[IBIS ver]   3.2
[File name]   sprm202c.ibs
[File Rev]   1.0
[Date]   August 11, 2005
[Source]   TI
[Disclaimer]   Please be aware that in the absence of a written agreement
|   Texas Instruments(TI) assumes no liability for:
|   (1) The accuracy of the IBIS models provided to your company
|   (2) The proper functioning of these Models in your design
|   or for any resulting applications
|   (3) Infringement of patents, copyrights or intellectual
|   property rights resulting from your use of these
|   models.
|   TI provides IBIS Models as a service to our customers and
|   therefore reserves the right to limit distribution of the
|   Models.
[Copyright]   Property of Texas Instruments Incorporated.
|   Unauthorized reproduction and/or distribution is strictly.
|   prohibited.
|   This product is protected under copyright law and trade
|   secret law as an unpublished work.
|   Created 2003,(C) Copyright 1999-2003,
|   Texas Instruments Incorporated., All Rights Reserved.
|   These commodities are under the U.S. Government
|   distribution license control. As such,they are not to be
|   re-exported without the prior approval of the U.S.
|   Department of Commerce.
[Notes]   See individual buffer models for additional notes.
|****** ****   ***** *****   ******  Package Model  ***************************
[Component]   DAVINCI_ZWT
[Manufacturer]  Texas Instruments
[Package]
|variable   typ   min   max
R_pkg   0.30489   0.23517194   0.41076
L_pkg   4.09242n   2.12433n   9.57717n
C_pkg   1.20919p   1.16455p   1.41723p
[Pin] signal_name   model_name   R_pin   L_pin   C_pin
K17  YI1_CCD1   BC1850BSHYPDFZ   0.27142   3.26611n   1.24171p
E11  GIOV3310_RXD3   BT3350BSHYPDFZP18_Z 0.26648   3.27345n   1.21648p
D8   SD_DATA0   BT3350BSHYPDFZP18_Z 0.26424   3.13901n   1.23471p
C11  GIOV338_RXD1   BT3350BSHYPDFZP18_Z 0.32683   4.77147n   1.21112p
E4   EMD4_DD4   BC1850BSHYPDFZ_PDZ  0.24370885  2.59914n   1.25295p
N19  CI7_CCD15_UARTRXD2   BC1850BSHYPDFZ   0.32265   4.61826n   1.18113p
N18  CI6_CCD1_UARTTXD2   BC1850BSHYPDFZ   0.30424   3.95206n   1.18245p
N17  CI5_CCD13_UARTCTS2   BC1850BSHYPDFZ   0.23966353  2.25930n   1.17595p
N15  CI3_CCD11   BC1850BSHYPDFZ   0.25136   2.72422n   1.21653p
M15  CI0_CCD8   BC1850BSHYPDFZ   0.23948995  2.24177n   1.1961p
N16  CI4_CCD12_UARTRTS2   BC1850BSHYPDFZ   0.32117   4.53767n   1.23269p
M17  CI2_CCD10   BC1850BSHYPDFZ   0.29397   3.52173n   1.18996p
M16  CI1_CCD9   BC1850BSHYPDFZ   0.29839   3.66820n   1.19339p
M19  PCLK   BC1850BSHYPDFZ_PDZ  0.32124   4.54005n   1.16939p
L19  VD   BC1850BSHYPDFZ_PDZ  0.32051   4.55204n   1.17582p
M18  HD   BC1850BSHYPDFZ_PDZ  0.30044   3.73376n   1.16728p
L18  YI7_CCD7   BC1850BSHYPDFZ   0.30158   3.82514n   1.17562p
L17  YI6_CCD6   BC1850BSHYPDFZ   0.24008563  2.27632n   1.175p
L16  YI5_CCD5   BC1850BSHYPDFZ   0.31818   4.44138n   1.22761p
L15  YI4_CCD4   BC1850BSHYPDFZ   0.25554   2.83961n   1.21082p
K19  YI3_CCD3   BC1850BSHYPDFZ   0.3193   4.49825n   1.17099p
K18  YI2_CCD2   BC1850BSHYPDFZ   0.30113   3.80508n   1.17045p
K16  YI0_CCD0   BC1850BSHYPDFZ   0.29716   3.67499n   1.19867p
E19  CLKOUT1_TIMIN_GPIO49   BC1850BSHYPDFZ_PDZ  0.34024   5.31946n   1.20264p
E15  YOUT4_R4_AEAW4   BC1850BSHYPDFZ   0.34642   5.54214n   1.30793p
E16  YOUT5_R5   BC1850BSHYPDFZ_PDZ  0.32347   4.68532n   1.28314p
D19  VCLK   BC1850BSHYPDFZ_PDZ  0.34898   5.65973n   1.2157p
C19  VPBECLK   BC1850BSHYPDFZ   0.35532   5.90192n   1.225p
B19  COUT6_G3   BC1850BSHYPDFZ_PDZ  0.36768   6.39976n   1.24506p
E18  YOUT7_R7   BC1850BSHYPDFZ_PDZ  0.30638   4.04896n   1.24212p
E17  YOUT6_R6   BC1850BSHYPDFZ_PDZ  0.30907   4.16196n   1.28916p
D15  YOUT0_G5_AEAW0   BC1850BSHYPDFZ   0.3463   5.62598n   1.37049p
D16  YOUT1_G6_AEAW1   BC1850BSHYPDFZ   0.31601   5.21148n   1.33301p
C16  COUT7_G4   BC1850BSHYPDFZ_PDZ  0.3081   4.99577n   1.34461p
D18  YOUT3_R3_AEAW3   BC1850BSHYPDFZ   0.31075   4.22512n   1.2403p
C18  VSYNC   BC1850BSHYPDFZ   0.31724   4.48625n   1.23593p
B18  COUT5_G2   BC1850BSHYPDFZ_PDZ  0.33021   4.96230n   1.23197p
C17  HSYNC   BC1850BSHYPDFZ   0.30581   4.10873n   1.2456p
D17  YOUT2_G7_AEAW2   BC1850BSHYPDFZ   0.30617   4.87215n   1.28815p
B17  COUT3_B6_DSPBT   BC1850BSHYPDFZ   0.329   4.61176n   1.20617p
A18  COUT4_B7   BC1850BSHYPDFZ_PDZ  0.33688   4.93706n   1.20091p
B16  COUT1_B4_BTSEL1   BC1850BSHYPDFZ   0.30834   3.87063n   1.19717p
A17  COUT2_B5_EMWIDTH   BC1850BSHYPDFZ   0.32513   4.53204n   1.19667p
C15  PWM0_GPIO45   BC1850BSHYPDFZ_PDZ  0.25161   2.59187n   1.20447p
B15  PWM1_R2_GPIO46   BC1850BSHYPDFZ_PDZ  0.31665   4.23770n   1.19062p
E14  GPIO5_G1   BC1850BSHYPDFZ_PDZ  0.25976   2.88215n   1.22562p
A16  COUT0_B3_BTSEL0   BC1850BSHYPDFZ   0.33512   4.91629n   1.18803p
P5   EMA18_GIO13_VLNQRXD1   BC1850BSHYPDFZ_PDZ  0.25928   3.04090n   1.26652p
R5   EMA16_GIO15_VLNQRXD2   BC1850BSHYPDFZ_PDZ  0.2672   3.33832n   1.25638p
T2   EMCS4_GIO9_VLNQSCRUN   BC1850BSHYPDFZ_PDZ  0.29472   3.50721n   1.18161p
T1   EMCS5_GIO8_VLNQCLOCK   BC1850BSHYPDFZ_PDZ  0.30976   4.10843n   1.1798p
T3   EMA21_GIO10_VLNQTXD0   BC1850BSHYPDFZ_PDZ  0.29934   3.81398n   1.21837p
R4   EMA19_GIO12_VLNQTXD1   BC1850BSHYPDFZ_PDZ  0.30272   3.86488n   1.21797p
N4   EMA13_GPIO18   BC1850BSHYPDFZ_PDZ  0.23736136  2.17244n   1.21241p
R3   EMA20_GIO11_VLNQRXD0   BC1850BSHYPDFZ_PDZ  0.29279   3.54781n   1.20942p
R2   EMA17_GIO14_VLNQTXD2   BC1850BSHYPDFZ_PDZ  0.30435   3.91825n   1.18246p
P3   EMA15_GIO16_VLNQTXD3   BC1850BSHYPDFZ_PDZ  0.29342   3.47425n   1.20306p
P4   EMA14_GIO17_VLNQRXD3   BC1850BSHYPDFZ_PDZ  0.29742   3.72080n   1.22221p
R1   EMA12_GPIO19   BC1850BSHYPDFZ_PDZ  0.33141   4.91831n   1.18807p
P1   EMA10_GPIO21   BC1850BSHYPDFZ_PDZ  0.32107   4.51855n   1.17303p
P2   EMA11_GPIO20   BC1850BSHYPDFZ_PDZ  0.30527   3.92717n   1.1797p
N3   EMA8_GPIO23   BC1850BSHYPDFZ_PDZ  0.29205   3.40450n   1.18847p
L4   RESETN   IC18SHYPUFZ   0.24060459  2.27896n   1.19435p
M4   EMA9_GPIO22   BC1850BSHYPDFZ_PDZ  0.23754022  2.16867n   1.17725p
N1   EMA6_GPIO25   BC1850BSHYPDFZ_PDZ  0.32162   4.52466n   1.17019p
K1   CLKOUT0_GPIO48   BC1850BSHYPDFZ_PDZ  0.30266   3.85884n   1.17499p
L1   CLKIN   IOSCHF18SHY   0.31844   4.39342n   1.16471p
K4   EMA4_GPIO27   BC1850BSHYPDFZ_PDZ  0.32093   4.55345n   1.22883p
J5   GPIO50_ATACS0   BC1850BSHYPDFZ_PDZ  0.25488   2.84503n   1.21689p
J4   EMA0_DA2_GPIO53   BC1850BSHYPDFZ_PDZ  0.23939151  2.29806n   1.18231p
J3   EMBA0_DA0   BC1850BSHYPDFZ_PDZ  0.2359258   2.13113n   1.17721p
K3   EMA5_GPIO26   BC1850BSHYPDFZ_PDZ  0.29597   3.55241n   1.18676p
K2   EMA3_GPIO28   BC1850BSHYPDFZ_PDZ  0.29881   3.67469n   1.16455p
J1   EMA2   BC1850BSHYPDFZ_PDZ  0.3178   4.41430n   1.16743p
H3   DMACK_UARTTXD1   BC1850BSHYPDFZ_PDZ  0.28904   3.34897n   1.19571p
H1   GPIO51_ATACS1   BC1850BSHYPDFZ_PDZ  0.31476   4.31632n   1.16847p
J2   EMA1   BC1850BSHYPDFZ_PDZ  0.29951   3.72938n   1.16729p
H2   EMBA1_DA1_GPIO52   BC1850BSHYPDFZ_PDZ  0.30016   3.76002n   1.16876p
G1   DMARQ_UARTRXD1   BC1850BSHYPDFZ   0.32209   4.59886n   1.17782p
D14  GPIO38_R1   BC1850BSHYPDFZ_PDZ  0.24943373  2.49462n   1.19177p
E13  GPIO1_CWE   BC1850BSHYPDFZ_PDZ  0.24702782  2.38582n   1.20009p
D13  GPIO2_G0   BC1850BSHYPDFZ_PDZ  0.24580039  2.35534n   1.19321p
D12  GIOV334_TXD1   BT3350BSHYPDFZP18_Z 0.25534   2.76733n   1.21955p
E12  GIOV337_RXD0   BT3350BSHYPDFZP18_Z 0.25098   2.49201n   1.21562p
E10  GIOV3315_MDIO   BT3350BSHYPDFZP18_Z 0.25609   2.68714n   1.21016p
E9   SD_DATA1   BT3350BSHYPDFZP18_Z 0.26906   3.20966n   1.23725p
A15  PWM2_B2_GPIO47   BC1850BSHYPDFZ_PDZ  0.33245   4.82511n   1.18357p
A14  GPIO6_B1   BC1850BSHYPDFZ_PDZ  0.33354   4.86754n   1.18579p
B14  GPIO4_R0_CFIELD   BC1850BSHYPDFZ_PDZ  0.31277   4.12134n   1.1868p
C14  GPIO3_B0_LCDFIELD   BC1850BSHYPDFZ_PDZ  0.29883   3.54970n   1.19368p
C13  GPIO0_LCDOE   BC1850BSHYPDFZ_PDZ  0.30633   3.83629n   1.20463p
C12 GIOV336_TXD3   BT3350BSHYPDFZP18_Z 0.30666   3.80383n   1.20363p
A11 GIOV335_TXD2   BT3350BSHYPDFZP18_Z 0.33469   4.95163n   1.19018p
A12 GIOV332_COL   BT3350BSHYPDFZP18_Z 0.32801   4.64818n   1.17868p
A13 GIOV331_TXCLK   BT3350BSHYPDFZP18_Z 0.31242   4.05710n   1.17723p
B13 GIOV330_TXEN   BT3350BSHYPDFZP18_Z 0.30624   3.82421n   1.17796p
B12 GIOV333_TXD0   BT3350BSHYPDFZP18_Z 0.31117   4.04273n   1.18423p
B11 GIOV339_RXD2   BT3350BSHYPDFZP18_Z 0.31218   4.00065n   1.17507p
A10 GIOV3311_RXCLK   BT3350BSHYPDFZP18_Z 0.33193   4.78827n   1.18217p
D11 GIOV3312_RXDV   BT3350BSHYPDFZP18_Z 0.31026   3.93739n   1.20497p
D10 GIOV3313_RXER   BT3350BSHYPDFZP18_Z 0.31235   4.09340n   1.21604p
C10 GIOV3314_CRS   BT3350BSHYPDFZP18_Z 0.31221   3.99279n   1.2065p
B10 GIOV3316_MDCLK   BT3350BSHYPDFZP18_Z 0.31256   4.00376n   1.17687p
C9  SD_DATA3   BT3350BSHYPDFZP18_Z 0.31135   3.97934n   1.20841p
A9  SD_CLK   BT3350BSHYPDFZP18_Z 0.33142   4.72337n   1.17817p
B9  SD_CMD   BT3350BSHYPDFZP18_Z 0.31656   4.20830n   1.18471p
D9  SD_DATA2   BT3350BSHYPDFZP18_Z 0.31824   4.24185n   1.21905p
C8  FSX_GIO31   BC1850BSHYPDFZ_PDZ  0.31499   4.10649n   1.21449p
B8  CLKX_GPIO29   BC1850BSHYPDFZ_PDZ  0.31718   4.24766n   1.18779p
A8  CLKR_GPIO30   BC1850BSHYPDFZ_PDZ  0.32026   4.30407n   1.18253p
F5  EMD2_DD2   BC1850BSHYPDFZ_PDZ  0.24446141  2.54036n   1.26565p
D7  NTRST   IC18SHYPDFZ   0.25102   2.57722n   1.20656p
D6  EMU0   BC1850BSHYPUFZ   0.26369   3.00542n   1.22142p
E6  TMS   IC18SHYPUFZ   0.26016   2.89933n   1.23079p
D5  UARTRXD0_GPIO35   BC1850BSHYPDFZ_PDZ  0.32087   4.37168n   1.23559p
C3  GPIO7   BC1850BSHYPDFZ_PDZ  0.28444   3.81897n   1.26078p
H5  EMD14_DD14   BC1850BSHYPDFZ_PDZ  0.25134   2.74799n   1.2613p
G5  EMD10_DD10   BC1850BSHYPDFZ_PDZ  0.24763525  2.62779n   1.25179p
H4  EMOE_DIOR   BC1850BSHYPDFZ_PDZ  0.23517194  2.12433n   1.183p
G3  EMRNW_INTRQ   BC1850BSHYPDFZ_PDZ  0.24110686  2.36803n   1.22429p
F4  EMD6_DD6   BC1850BSHYPDFZ_PDZ  0.23553426  2.20052n   1.22333p
G2  EMWE_DIOW   BC1850BSHYPDFZ_PDZ  0.3026   3.92018n   1.18023p
F1  EMWAIT_IORDY   BC1850BSHYPUFZ   0.32084   4.57333n   1.17696p
E1  EMD15_DD15   BC1850BSHYPDFZ_PDZ  0.33258   5.06281n   1.19705p
F2  EMD13_DD13   BC1850BSHYPDFZ_PDZ  0.30858   4.20967n   1.20886p
D1  EMD12_DD12   BC1850BSHYPDFZ_PDZ  0.34172   5.41604n   1.2124p
G4  EMD11_DD11   BC1850BSHYPDFZ_PDZ  0.29109   3.46731n   1.23452p
F3  EMD8_DD8   BC1850BSHYPDFZ_PDZ  0.28411   3.21952n   1.22681p
E2  EMD9_DD9   BC1850BSHYPDFZ_PDZ  0.30321   3.93813n   1.21141p
C1  EMD7_DD7   BC1850BSHYPDFZ_PDZ  0.34316   5.47607n   1.21459p
D2  EMD5_DD5   BC1850BSHYPDFZ_PDZ  0.30837   4.15257n   1.21424p
E5  EMD0_DD0   BC1850BSHYPDFZ_PDZ  0.23865047  2.31435n   1.2451p
E3  EMD3_DD3   BC1850BSHYPDFZ_PDZ  0.28366   3.21871n   1.22369p
D3  EMD1_DD1   BC1850BSHYPDFZ_PDZ  0.2921   3.60704n   1.24282p
C7  FSR_GPIO32   BC1850BSHYPDFZ_PDZ  0.31555   4.22094n   1.21883p
A7  DR_GPIO34   BC1850BSHYPDFZ_PDZ  0.32996   4.67616n   1.17937p
C6  EMU1   BC1850BSHYPUFZ   0.3118   4.01559n   1.20949p
B7  DX_GPIO33   BC1850BSHYPDFZ_PDZ  0.31643   4.22763n   1.18564p
A6  TCK   IC18SHYPUFZ   0.3335   4.85058n   1.1798p
B5  TDO   OC1850BSFZ   0.32041   4.41194n   1.19295p
A5  TDI   IC18SHYPUFZ   0.33719   4.99894n   1.18952p
C4  SCL_GPIO43   BC1850BSHYPDFZ_PDZ  0.31456   4.20146n   1.23233p
C5  UARTTXD0_GPIO38   BC1850BSHYPDFZ_PDZ  0.30441   3.82552n   1.21979p
B4  SDA_GPIO44   BC1850BSHYPDFZ_PDZ  0.32308   4.45433n   1.19164p
B6  RTCK   OC1850BSFZ   0.31193   4.03099n   1.17724p
A3  SPICLK_GPIO39   BC1850BSHYPDFZ_PDZ  0.33139   4.77785n   1.19765p
B3  SPIDI_GPIO40   BC1850BSHYPDFZ_PDZ  0.32391   4.48887n   1.20374p
A4  SPIEN0_GPIO37   BC1850BSHYPDFZ_PDZ  0.34182   5.15828n   1.19449p
B2  SPIEN1_GPIO42   BC1850BSHYPDFZ_PDZ  0.33542   4.91202n   1.21886p
A2  SPIDO_GPIO41   BC1850BSHYPDFZ_PDZ  0.34148   5.16190n   1.21506p
B1  EM_CS3   BC1850BSHYPDFZ_PDZ  0.34927   5.38565n   1.22986p
C2  EM_CS2   BC1850BSHYPDFZ_PDZ  0.3251   4.50591n   1.22482p
N2  EMA7_GPIO24   BC1850BSHYPDFZ_PDZ  0.30209   3.80241n   1.17344p
|****** ****   ***** *****   ******  Buffer Models  ***************************
|   Component BC1850BSHYPDFZ
|[Notes]   Driver/Receiver, CMOS, 1.8 V, 50 ohms, Fnom < 100 MHz,
|   min-height, non-failsafe, hysteresis, pulldown, with HHV
[Component]   BC1850BSHYPDFZ
[Manufacturer]   Texas Instruments.
[Package]
| variable   typ   min   max
R_pkg   0.000   0.000   0.000
L_pkg   0.000H   0.000H   0.000H
C_pkg   0.000F   0.000F   0.000F
[Pin]  signal_name   model_name   R_pin   L_pin   C_pin
1   PAD   BC1850BSHYPDFZ
|2   A   (input)
|3   GZ   (Driver enable)
|4   HHV   (force Z)
|5   PI   (pulldown Inhibit)
|6   Y   (receiver output)
|7   VDD   (1.2V core supply)
8   VDDS   POWER
9   VSS   GND
10   VSSS   GND
[Model Selector]   BC1850BSHYPDFZ
BC1850BSHYPDFZ_1P8PD   Cell operated at VDDS=1.8V(nom) with pulldown "on"
BC1850BSHYPDFZ_PDZ   Cell operated at VDDS=1.8V(nom) with pulldown "off"
|   Component BC1850BSHYPUFZ
|[Notes]   Driver/Receiver, CMOS, 1.8 V, 50 ohms, Fnom < 100 MHz,
|   min-height, non-failsafe, hysteresis, pull-up, with HHV
[Component]   BC1850BSHYPUFZ
[Manufacturer]   Texas Instruments.
[Package]
| variable   typ   min   max
R_pkg   0.000   0.000   0.000
L_pkg   0.000H   0.000H   0.000H
C_pkg   0.000F   0.000F   0.000F
[Pin]  signal_name   model_name   R_pin   L_pin   C_pin
1   PAD   BC1850BSHYPUFZ
|2   A   (input)
|3   GZ   (Driver enable)
|4   HHV   (force Z)
|5   PI   (pullup Inhibit)
|6   Y   (receiver output)
|7   VDD   (1.2V core supply)
8   VDDS   POWER
9   VSS   GND
10   VSSS   GND
[Model Selector]   BC1850BSHYPUFZ
BC1850BSHYPUFZ_PU   Cell operated at VDDS=1.8V(nom) with Pullup "on"
BC1850BSHYPUFZ_PUZ   Cell operated at VDDS=1.8V(nom) with Pullup "off"
|   Component BC1850CSHYPDFZ
|[Notes]   Driver/Receiver, CMOS, 1.8 V, 50 ohms, Fnom < 150 MHz,
|   min-height, non-failsafe,hysteresis, pulldown, with HHV
[Component]   BC1850CSHYPDFZ
[Manufacturer]   Texas Instruments.
[Package]
| variable   typ   min   max
R_pkg   0.000   0.000   0.000
L_pkg   0.000H   0.000H   0.000H
C_pkg   0.000F   0.000F   0.000F
[Pin]  signal_name   model_name   R_pin   L_pin   C_pin
1   PAD   BC1850CSHYPDFZ
8   VDDS   POWER
9   VSS   GND
10   VSSS   GND
[Model Selector]   BC1850CSHYPDFZ
BC1850CSHYPDFZ_1P8PD   Cell operated at VDDS=1.8V(nom) with pulldown "on"
BC1850CSHYPDFZ_PDZ   Cell operated at VDDS=1.8V(nom) with pulldown "off"
|   Component BT3350BSHYPDFZP18
|[Notes]   Driver/Receiver, TTL, 3.3 V, 50 ohms, Fnom < 100 Mhz,
|   min-height , non-failsafe, hystersis, pull-down
[Component]   BT3350BSHYPDFZP18
[Manufacturer]   Texas Instruments.
[Package]
| variable   typ   min   max
R_pkg   0.000   0.000   0.000
L_pkg   0.000H   0.000H   0.000H
C_pkg   0.000F   0.000F   0.000F
[Pin]  signal_name   model_name   R_pin   L_pin   C_pin
1   PAD   BT3350BSHYPDFZP18
|2   A   (input)
|3   GZ   (Driver enable)
|4   HHV   (Driver tristate)
|5   PI   (pulldown Inhibit)
|6   PWRDN   (low power mode control signal)
|7   Y   (receiver output)
|8   VDD   (1.2V core supply)
9   VDDS   POWER
10   VSS   GND
11   VSSS   GND
[Model Selector]   BT3350BSHYPDFZP18
BT3350BSHYPDFZP18_PD   Cell operated at VDDS=3.3V(nom) with Pulldown "on"
BT3350BSHYPDFZP18_Z   Cell operated at VDDS=3.3V(nom) with Pulldown "off"
|   Component IC18SHYPDFZ
|[Notes]   LVCMOS Receiver, 1.8V, min-height, pullup, HHV control
[Component]   IC18SHYPDFZ
[Manufacturer]   TI
[Package]
| variable   typ   min   max
R_pkg   0.000   0.000   0.000
L_pkg   0.000H   0.000H   0.000H
C_pkg   0.000F   0.000F   0.000F
[Pin]  signal_name   model_name   R_pin   L_pin   C_pin
1   PAD   IC18SHYPDFZ
|2   PI   (Pulldown inhibit)
|3   HHV   (Force Z)
|4   Y   (receiver output)
|5   VDD   (1.2V core supply)
6   VDDS   POWER
7   VSS   GND
[Model Selector]   IC18SHYPDFZ
IC18SHYPDFZ_1P8PD reflects VDDS=1.8V(typ) operation, Pulldown "on"
IC18SHYPDFZ_1P8PDZ reflects VDDS=1.8V(typ) operation, Pulldown "off"
|   Component IC18SHYPUFZ
|[Notes]   LVCMOS Receiver, 1.8V, min-height, pullup, HHV control
[Component]   IC18SHYPUFZ
[Manufacturer]   TI
[Package]
| variable   typ   min   max
R_pkg   0.000   0.000   0.000
L_pkg   0.000H   0.000H   0.000H
C_pkg   0.000F   0.000F   0.000F
[Pin]  signal_name   model_name   R_pin   L_pin   C_pin
1   PAD   IC18SHYPUFZ
|2   PI   (Pullup inhibit)
|3   HHV   (Force Z)
|4   Y   (receiver output)
|5   VDD   (1.2V core supply)
6   VDDS   POWER
7   VSS   GND
[Model Selector]   IC18SHYPUFZ
IC18SHYPUFZ_1P8PU reflects VDDS=1.8V(typ) operation, Pullup "on"
IC18SHYPUFZ_1P8PUZ reflects VDDS=1.8V(typ) operation, Pullup "off"
|   Component OC1850BSFZ
|[Notes]   Driver, CMOS, 1.8 V, 50 ohms, Fnom < 100 MHz, min-height,
|   non-failsafe, with HHV
[Component]   OC1850BSFZ
[Manufacturer]   Texas Instruments.
[Package]
| variable   typ   min   max
R_pkg   0.000   0.000   0.000
L_pkg   0.000H   0.000H   0.000H
C_pkg   0.000F   0.000F   0.000F
[Pin]  signal_name   model_name   R_pin   L_pin   C_pin
1   PAD   OC1850BSFZ
| 2   A   (Driver input)
| 3   GZ   (Driver enable)
| 4   HHV   (force Z)
5   VDDS   POWER
| 6   VDD   (1.2V core supply)
7   VSSS   GND
8   VSS   GND
|   Component IOSCHF18SHY
[Component]   IOSCHF18SHY
[Manufacturer]   Texas Instruments
[Package]
|   typ   min   max
R_pkg   0   0   0
L_pkg   0   0   0
C_pkg   0   0   0
[Pin]   signal_name   model_name   R_pin   L_pin   C_pin
   1   A   IOSCHF18SHY   0   0   0
| Models and submodels in the file (14): BC1850BSHYPDFZ_1P8PD (I/O), BC1850BSHYPDFZ_PDZ (I/O), BC1850BSHYPUFZ_PU (I/O), BC1850BSHYPUFZ_PUZ (I/O), BC1850CSHYPDFZ_1P8PD (I/O), BC1850CSHYPDFZ_PDZ (I/O), BT3350BSHYPDFZP18_PD (I/O), BT3350BSHYPDFZP18_Z (I/O), IC18SHYPDFZ_1P8PD (Input), IC18SHYPDFZ_1P8PDZ (Input), IC18SHYPUFZ_1P8PU (Input), IC18SHYPUFZ_1P8PUZ (Input), OC1850BSFZ (3-state), IOSCHF18SHY (Input)
